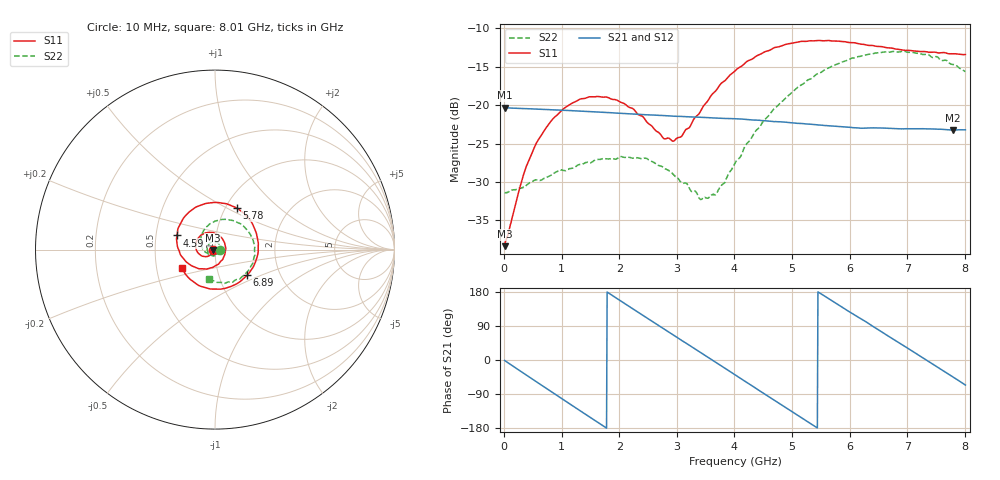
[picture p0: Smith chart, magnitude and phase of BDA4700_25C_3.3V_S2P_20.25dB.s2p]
!Agilent Technologies,E5071B,MY42404982,A.09.10
!Date: Mon Oct 20 18:11:33 2025
!Data & Calibration Information:
!Freq	S11:SOLT2(ON)	S21:SOLT2(ON)	S12:SOLT2(ON)	S22:SOLT2(ON)
# Hz S RI R 50
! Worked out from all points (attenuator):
!   801 points, 10 MHz to 8.01 GHz, reference 50 ohm
!   highest |S21| = -20.32 dB at 10 MHz (marker M1); lowest = -23.3 dB at 7.8 GHz (marker M2)
!   lowest |S11| = -38.4 dB at 10 MHz (marker M3), VSWR 1.02, Z = 48.8 - j0.152 ohm
!   |S11| at or under -10 dB: start of sweep to end of sweep
!   |S22| runs from -32.3 to -13.0 dB; largest |S21 - S12| = 0.0011
!   S11 on the Smith chart (normalised r, x): 10 MHz: 0.98, -0.00; 4.59 GHz: 0.64, +0.11; 5.78 GHz: 1.12, +0.56; 6.89 GHz: 1.37, -0.41; 8.01 GHz: 0.67, -0.15
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1e7  -0.012 -0.00155  0.0963 -0.00205  0.0962 -0.00212  0.0269 -0.000811
3.4e8  -0.0231 -0.0268  0.0777 -0.0544  0.0777 -0.0545  0.0232 -0.0179
5.7e8  -0.0425 -0.0384  0.0495 -0.0801  0.0494 -0.0801  0.0149 -0.0291
8.7e8  -0.0755 -0.0342  0.0023 -0.093  0.00239 -0.0931  -0.00643 -0.0355
1.35e9  -0.1085 0.0183  -0.0665 -0.0625  -0.0665 -0.0626  -0.037 -0.018
1.96e9  -0.0552 0.0925  -0.0845 0.0269  -0.0846 0.0269  -0.035 0.0281
2.45e9  0.0256 0.0762  -0.0351 0.079  -0.0352 0.0791  -0.00209 0.0452
2.68e9  0.0522 0.041  -0.002 0.0857  -0.00217 0.0857  0.0143 0.0379
2.96e9  0.0569 -0.0147  0.037 0.076  0.037 0.0759  0.0269 0.022
3.43e9  -0.00418 -0.0941  0.0792 0.0257  0.0793 0.0257  0.0197 -0.0143
3.69e9  -0.0658 -0.107  0.0816 -0.0107  0.0817 -0.0109  0.000553 -0.0264
4.01e9  -0.1468 -0.0789  0.0633 -0.0513  0.0634 -0.0511  -0.0324 -0.0264
4.59e9  -0.2114 0.0788  -0.00862 -0.0782  -0.00843 -0.0783  -0.0784 0.0329
4.94e9  -0.1659 0.1877  -0.0501 -0.0586  -0.0499 -0.0589  -0.071 0.0911
5.35e9  -0.0383 0.2588  -0.0739 -0.0123  -0.0738 -0.0127  -0.0154 0.1489
5.78e9  0.1198 0.232  -0.0618 0.0385  -0.0617 0.0384  0.0799 0.166
6.24e9  0.2289 0.0962  -0.0182 0.0684  -0.0171 0.0686  0.1801 0.1069
6.68e9  0.2238 -0.0731  0.0328 0.0625  0.033 0.0624  0.2207 -0.0027
6.89e9  0.1798 -0.142  0.0517 0.0471  0.0519 0.0468  0.2138 -0.0627
7.33e9  0.0295 -0.2203  0.07 -0.000157  0.0701 -0.00016  0.1424 -0.1598
7.8e9  -0.1397 -0.1647  0.0483 -0.049  0.0482 -0.0492  0.0167 -0.1828
8.01e9  -0.1864 -0.1038  0.028 -0.0631  0.0282 -0.063  -0.0331 -0.1615
